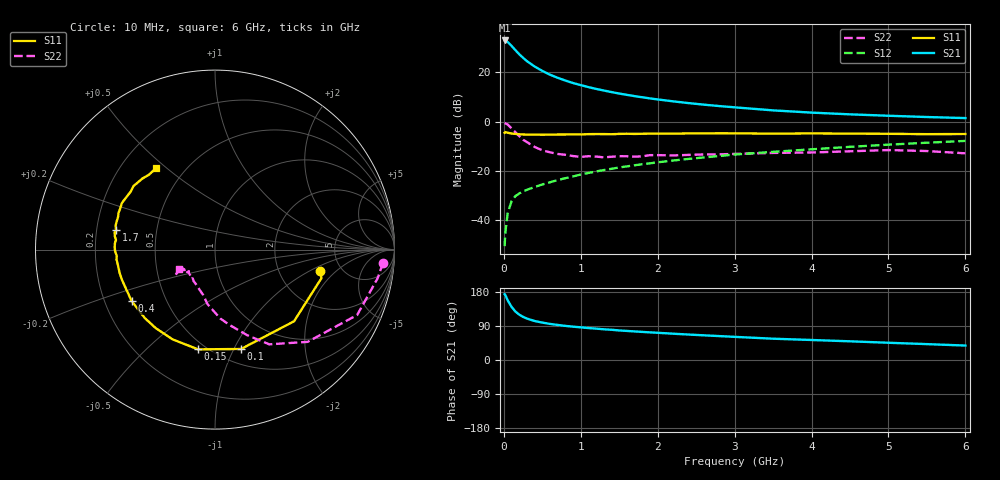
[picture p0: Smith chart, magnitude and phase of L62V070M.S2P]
!  INFINEON TECHNOLOGIES Small Signal Semiconductors
! BFR380L3 , Si-NPN RF-Transistor in TSLP-3-1
!  Vce=2 V,  Ic=70 mA
! Common Emitter S-Parameters:  07. March 2005
#  GHz  S  MA  R  50
! f  S11  S21  S12  S22
! GHz  Mag  Ang  Mag  Ang  Mag  Ang  Mag  Ang
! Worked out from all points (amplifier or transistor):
!   36 points, 10 MHz to 6 GHz, reference 50 ohm
!   highest |S21| = 32.9 dB at 10 MHz (marker M1)
!   |S21| within 3 dB of that: start of sweep to 123.6 MHz
!   unconditionally stable (mu >= 1): 1.257 GHz to 4.961 GHz
!   at 250 MHz: K = 0.52, MSG = 27.0 dB, |S12| = -28.3 dB
!   at 1.4 GHz: K = 1.02, MAG = 14.7 dB, |S12| = -19.1 dB
!   at 6 GHz: K = 0.98, MSG = 4.6 dB, |S12| = -7.8 dB
!   S11 on the Smith chart (normalised r, x): 10 MHz: 3.44, -1.27; 100 MHz: 0.65, -1.07; 150 MHz: 0.45, -0.74; 400 MHz: 0.32, -0.26; 1.7 GHz: 0.28, +0.09; 6 GHz: 0.35, +0.46
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0.01  0.5954 -11.5  43.92 173.8  0.003 74.7  0.9391 -4.5
0.02  0.6142 -15.0  43.47 171.1  0.0057 78.3  0.92 -10.0
0.05  0.5945 -42.2  40.87 157.6  0.0141 72.9  0.8719 -24.7
0.1  0.5723 -75.3  34.16 140.2  0.0243 61.9  0.7283 -44.9
0.15  0.5638 -99.6  27.99 127.9  0.0309 54.2  0.6082 -60.2
0.2  0.5531 -115.2  23.12 119.7  0.035 53.7  0.5086 -69.5
0.25  0.548 -127.2  19.56 113.8  0.0386 50.9  0.4289 -78.9
0.3  0.5463 -135.8  16.77 109.3  0.0415 51.9  0.3844 -85.7
0.4  0.5456 -148.3  13.05 102.9  0.0474 53.3  0.3069 -97.8
0.5  0.5418 -156.3  10.63 98.7  0.0532 55.2  0.2617 -104.5
0.6  0.5452 -162.1  8.9 95.2  0.0591 57.6  0.2388 -111.3
0.7  0.5472 -166.4  7.704 92.5  0.0654 59.4  0.2211 -118.2
0.9  0.5516 -174.4  6.03 88.0  0.0775 62.4  0.2004 -128.6
1.1  0.5565 -179.1  4.986 84.3  0.0911 64.0  0.1991 -133.2
1.4  0.5543 174.5  3.955 79.8  0.1106 65.3  0.1941 -139.3
1.7  0.5621 168.8  3.279 75.4  0.1305 65.9  0.1949 -146.5
2.2  0.5697 161.5  2.569 69.4  0.1628 66.1  0.2062 -146.9
2.8  0.5798 153.7  2.062 63.1  0.2008 65.8  0.217 -151.4
3.5  0.5699 145.5  1.686 56.2  0.2438 63.6  0.2319 -149.6
4.5  0.5707 139.3  1.401 49.3  0.3081 61.5  0.2502 -148.3
5.5  0.556 131.3  1.237 41.9  0.3734 57.5  0.2532 -148.0
6  0.5604 126.1  1.177 38.1  0.4062 55.2  0.2276 -151.2
